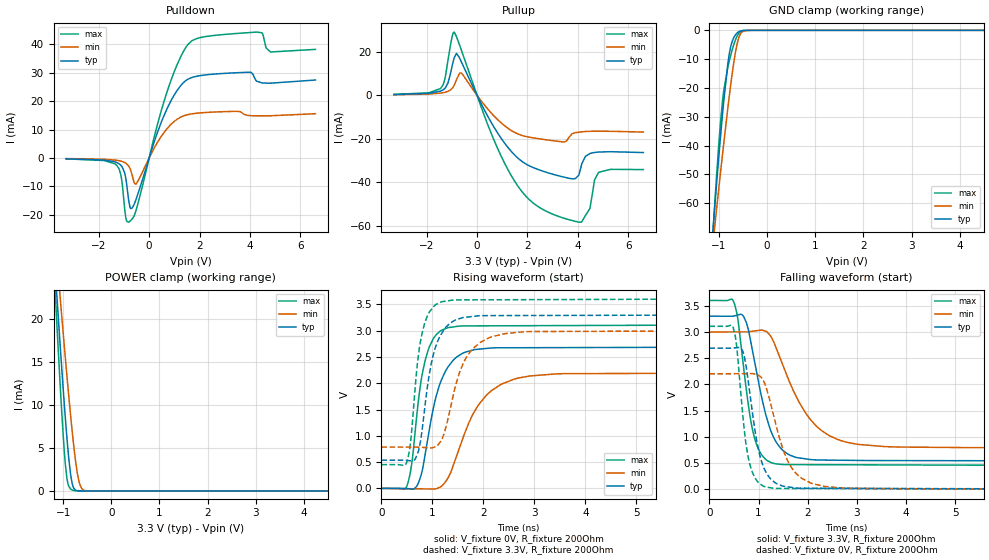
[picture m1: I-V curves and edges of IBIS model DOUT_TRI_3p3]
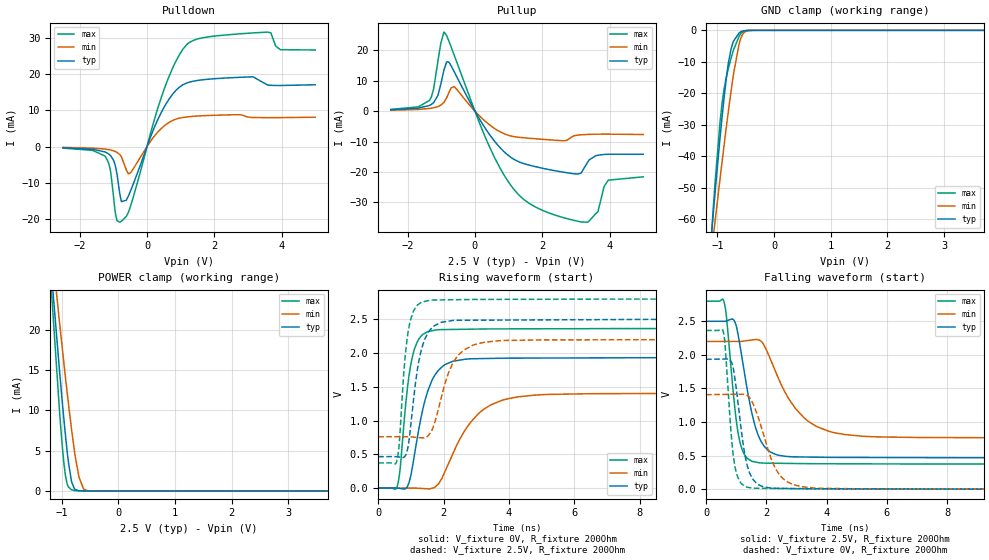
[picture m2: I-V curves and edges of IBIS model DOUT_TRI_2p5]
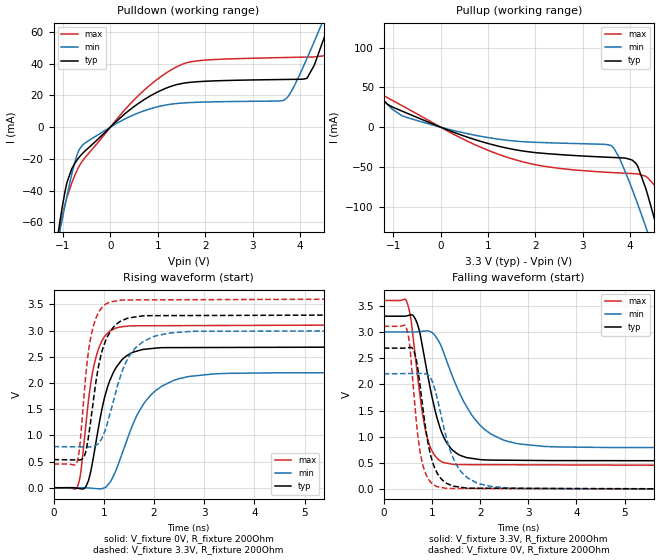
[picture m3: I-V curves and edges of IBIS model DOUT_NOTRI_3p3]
|Texas Instruments Incorporated
| Marketing part#   Digital Voltage Range   Package-type   #pins
| ADS1287D   2.2V - 3.6V   VQFN   32
[IBIS Ver]   4.1
[File name]   ads1287d.ibs
[File Rev]   1.0
[Date]   03/20/2017
[Source]
| Texas Instruments Incorporated.
| 12500 TI Blvd
| Dallas, TX -75243
[Notes]   Revision History:
| Rev 1.0: 03/20/2017
| - Initial version of the model
| - Model generated from simulations in TISPICE
| - C_comp although listed in numerical order of value are
|   obtained from varying PVT conditions. For PVT conditions for
|   each specific value refer the buffer description under
|   respective [Model]. IBIS model user is responsible for using
|   appropriate C_comp to simulate for Signal Integrity.
| - Warnings regarding combined Non-monotonicity of various models have been
|   reviewd and considered minor and can be ignored.
| - Model names with a trailing _2p5 contain the model for
|   2.5V operation. Model names with a trailing _3p3 contain the model
|   for 3.3V operation.
[Disclaimer]
| This model is designed as an aid for customers of Texas Instruments.
| TI and its licensors and suppliers make no warranties, either expressed
| or implied, with respect to this  model, including the warranties of
| merchantability or fitness for a particular purpose. The model is
| provided solely on an "as is" basis. The entire risk as to its quality
| and performance is with the customer.
[Copyright]
 (C) Copyright 2016 Texas Instruments Incorporated.All rights reserved.
|   Device
[Component]  ADS1287D
[Manufacturer]   TI
[Package]
| variable   typ   min   max
R_pkg   0.01   0.008   0.012
L_pkg   0.1nH   0.08nH   0.12nH
C_pkg   0.1pF   0.08pF   0.12pF
[Pin]  signal_name   model_name   R_pin   L_pin   C_pin
1   DRDY2\   DOUT_NOTRI   NA   NA   NA
2   DOUT   DOUT_TRI   NA   NA   NA
3   DIN   DIN   NA   NA   NA
4   CS1\   DIN   NA   NA   NA
5   CS2\   DIN   NA   NA   NA
6   SYNC   DIN   NA   NA   NA
7   TCP1   DIO   NA   NA   NA
8   TCP2   DIO   NA   NA   NA
9   CAPN1   NC   NA   NA   NA
10   CAPP1   NC   NA   NA   NA
11   CAPN2   NC   NA   NA   NA
12   CAPP2   NC   NA   NA   NA
13   TCR1   NC   NA   NA   NA
14   TCR2   NC   NA   NA   NA
15   AINP1   NC   NA   NA   NA
16   AINN1   NC   NA   NA   NA
17   AINP2   NC   NA   NA   NA
18   AINN2   NC   NA   NA   NA
19   AVDD   POWER   NA   NA   NA
20   AVSS   GND   NA   NA   NA
21   REFN   NC   NA   NA   NA
22   REFP   NC   NA   NA   NA
23   PWDN1\   DIN   NA   NA   NA
24   PWDN2\   DIN   NA   NA   NA
25   RESET\   DIN   NA   NA   NA
26   DVDD   POWER   NA   NA   NA
27   DGND   GND   NA   NA   NA
28   BYPAS1   NC   NA   NA   NA
29   BYPAS2   NC   NA   NA   NA
30   CLK   DIN_PD   NA   NA   NA
31   SCLK   DIN_PD   NA   NA   NA
32   DRDY1\   DOUT_NOTRI   NA   NA   NA
|   Model Selectors
[Model Selector]  DIN
DIN_3p3  input buffer at 3.3V operation.
DIN_2p5  input buffer at 2.5V operation.
[Model Selector]  DIN_PD
DIN_PD_3p3  input buffer at 3.3V operation.
DIN_PD_2p5  input buffer at 2.5V operation.
[Model Selector]  DIO
DIO_3p3  output buffer at 3.3V operation.
DIO_2p5  output buffer at 2.5V operation.
[Model Selector]  DOUT_TRI
DOUT_TRI_3p3  output buffer at 3.3V operation.
DOUT_TRI_2p5  output buffer at 2.5V operation.
[Model Selector]  DOUT_NOTRI
DOUT_NOTRI_3p3  output buffer at 3.3V operation.
DOUT_NOTRI_2p5  output buffer at 2.5V operation.
| Models and submodels in the file (10): DOUT_TRI_3p3 (3-state), DOUT_TRI_2p5 (3-state), DOUT_NOTRI_3p3 (Output), DOUT_NOTRI_2p5 (Output), DIO_3p3 (I/O), DIO_2p5 (I/O), DIN_PD_3p3 (Input), DIN_PD_2p5 (Input), DIN_3p3 (Input), DIN_2p5 (Input)
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|   Model
[Model]   DOUT_TRI_3p3
Model_type   3-state
Polarity   Non-Inverting
Vmeas = 1.65
Vref = 0
Cref = 1pF
Rref = 100000
|   typ   min   max
C_comp   3.353pF   2.933pF   3.722pF
[Voltage Range]   3.3   3   3.6
[Temperature Range]   27   125   -40
[Pullup Reference]   3.3   3   3.6
[Pulldown Reference]   0   0   -0
[Power Clamp Reference]   3.3   3   3.6
[GND Clamp Reference]   0   0   0
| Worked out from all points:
|   slope of the pulldown table from 0 to 0.495 V, typ, clamps not added: 38.4 ohm
|   slope of the pullup table from 0 to 0.495 V, typ, clamps not added: 44.6 ohm
|   GND clamp passes 1 mA (typ) near -0.63 V on its own axis
|   POWER clamp passes 1 mA (typ) near -0.82 V on its own axis
|   falling waveform, V_fixture 3.3V, R_fixture 200Ohm: 20-80 % time 405ps typ, 736ps min, 275ps max; typ from 3.3 V to 0.537 V
|   rising waveform, V_fixture 0V, R_fixture 200Ohm: 20-80 % time 381ps typ, 640ps min, 259ps max; typ from 0 V to 2.69 V
|   rising waveform, V_fixture 3.3V, R_fixture 200Ohm: 20-80 % time 288ps typ, 429ps min, 211ps max; typ from 0.537 V to 3.3 V
|   falling waveform, V_fixture 0V, R_fixture 200Ohm: 20-80 % time 282ps typ, 440ps min, 207ps max; typ from 2.69 V to 0 V
[Pulldown]
|   Voltage   I(typ)   I(min)   I(max)
-3.3V     -275.6uA   -195.7uA   -299.2uA
-1.29V    -1.589mA   -812uA     -2.567mA
-1.112V   -2.674mA   -1.126mA   -6.407mA
-973.5mV  -5.243mA   -1.59mA    -17.68mA
-815.1mV  -14.85mA   -2.806mA   -22.59mA
-726mV    -17.84mA   -4.463mA   -21.94mA
-518.1mV  -14.5mA    -9.108mA   -18.41mA
709.5mV   17.33mA    10.32mA    23.26mA
1.68V     28.27mA    15.51mA    41.13mA
4.274V    27.01mA    14.85mA    44.32mA
4.818V    26.34mA    14.87mA    37.31mA
6.6V      27.45mA    15.59mA    38.23mA
[GND Clamp]
|   Voltage   I(typ)   I(min)   I(max)
-3.3V     -596mA     -481.9mA   -706.9mA
-1.191V   -83.7mA    -85.04mA   -87.73mA
-1.092V   -62.16mA   -68.77mA   -61.24mA
-1.063V   -55.89mA   -64.02mA   -53.64mA
-983.4mV  -39.78mA   -51.67mA   -34.99mA
-904.2mV  -25.08mA   -39.7mA    -21.25mA
-815.1mV  -11.44mA   -26.82mA   -12.68mA
-755.7mV  -5.637mA   -18.79mA   -8.611mA
-656.7mV  -1.555mA   -7.52mA    -3.281mA
-567.6mV  -310.1uA   -1.686mA   -686.5uA
-280.5mV  -30.52nA   -1.575uA   -574.7nA
6.6V      0A         0A         0A
[Pullup]
|   Voltage   I(typ)   I(min)   I(max)
-3.3V     367.9uA    267.7uA    426.7uA
-1.439V   1.996mA    1.043mA    3.259mA
-1.162V   5.477mA    1.816mA    15.57mA
-914.1mV  17.05mA    4.508mA    29.15mA
-617.1mV  15.27mA    10.17mA    20.63mA
986.7mV   -20.32mA   -13mA      -28.77mA
2.373V    -33.95mA   -19.86mA   -50.87mA
3.769V    -38.49mA   -17.71mA   -57.69mA
4.125V    -33.01mA   -16.86mA   -58.46mA
4.471V    -26.85mA   -16.59mA   -52.31mA
4.818V    -26.14mA   -16.53mA   -35.56mA
6.6V      -26.37mA   -16.92mA   -34.22mA
[POWER Clamp]
|   Voltage   I(typ)   I(min)   I(max)
-3.3V     222.9mA    184.2mA    273.8mA
-1.181V   27.13mA    30.69mA    24.94mA
-1.122V   22.01mA    26.62mA    18.54mA
-1.063V   17.02mA    22.61mA    12.42mA
-1.003V   12.21mA    18.66mA    6.83mA
-953.7mV  8.435mA    15.45mA    3.071mA
-904.2mV  5.034mA    12.34mA    929.6uA
-844.8mV  1.889mA    8.78mA     223.7uA
-805.2mV  702.8uA    6.57mA     94.47uA
-676.5mV  12.39uA    1.245mA    3.073uA
-528mV    121.8nA    27.64uA    0A
6.6V      0A         0A         0A
[Ramp]
R_load = 200
|   typ   min   max
dV/dt_r   1.61412/3.77044e-10   1.32022/6.35916e-10   1.86431/2.58199e-10
dV/dt_f   1.65772/4.03606e-10   1.32906/7.34637e-10   1.88895/2.74389e-10
[Falling Waveform]
V_fixture = 3.3V
V_fixture_min = 3V
V_fixture_max = 3.6V
R_fixture = 200Ohm
C_fixture = 0F
|   Time   V(typ)   V(min)   V(max)
0s        3.3V       3V         3.6V
490.8ps   3.301V     3V         3.583V
696.4ps   3.296V     3V         2.328V
829.8ps   2.875V     3.007V     1.381V
966.6ps   2.208V     3.024V     838.8mV
1.218ns   1.199V     2.954V     525.5mV
1.464ns   769.1mV    2.442V     471.8mV
2.281ns   555.1mV    1.118V     466.8mV
3.566ns   545.6mV    812.4mV    463.2mV
50ns      537.1mV    784.9mV    451.7mV
[Rising Waveform]
V_fixture = 0V
V_fixture_min = 0V
V_fixture_max = 0V
R_fixture = 200Ohm
C_fixture = 0F
|   Time   V(typ)   V(min)   V(max)
0s        -237.1nV   -255.9nV   -93.79nV
490.8ps   -2.67mV    -5.275mV   28.16mV
594.8ps   -11.92mV   -6.392mV   472.9mV
696.4ps   50.2mV     -7.484mV   1.418V
946.5ps   1.156V     -10.17mV   2.708V
1.172ns   2.054V     38.1mV     3.003V
1.525ns   2.53V      758.1mV    3.086V
2.164ns   2.67V      1.863V     3.091V
3.566ns   2.677V     2.182V     3.096V
50ns      2.69V      2.2V       3.107V
[Rising Waveform]
V_fixture = 3.3V
V_fixture_min = 3V
V_fixture_max = 3.6V
R_fixture = 200Ohm
C_fixture = 0F
|   Time   V(typ)   V(min)   V(max)
0s        537.1mV    784.9mV    451.7mV
490.8ps   533mV      785.1mV    486mV
574.3ps   525mV      785.2mV    912.4mV
666.4ps   562.7mV    785.2mV    1.975V
908.3ps   1.979V     773.8mV    3.295V
1.172ns   2.932V     906.5mV    3.544V
1.407ns   3.18V      1.765V     3.582V
1.802ns   3.271V     2.666V     3.585V
2.901ns   3.287V     2.982V     3.589V
50ns      3.3V       3V         3.6V
[Falling Waveform]
|Gnd
V_fixture = 0V
V_fixture_min = 0V
V_fixture_max = 0V
R_fixture = 200Ohm
C_fixture = 0F
|   Time   V(typ)   V(min)   V(max)
0s        2.69V      2.2V       3.107V
482ps     2.692V     2.203V     3.09V
553.5ps   2.699V     2.203V     2.744V
666.4ps   2.658V     2.203V     1.554V
873.1ps   1.484V     2.204V     326.2mV
1.052ns   558.8mV    2.137V     87.07mV
1.303ns   148.5mV    1.421V     16.29mV
1.767ns   21.14mV    296.3mV    13.28mV
2.791ns   15.52mV    19.55mV    11.12mV
50ns      -231.5nV   -246.5nV   -88.11nV
|   Model
[Model]   DOUT_TRI_2p5
Model_type   3-state
Polarity   Non-Inverting
Vmeas = 1.25
Vref = 0
Cref = 1pF
Rref = 100000
|   typ   min   max
C_comp   3.353pF   2.933pF   3.722pF
[Voltage Range]   2.5   2.2   2.8
[Temperature Range]   27   125   -40
[Pullup Reference]   2.5   2.2   2.8
[Pulldown Reference]   0   0   0
[Power Clamp Reference]   2.5   2.2   2.8
[GND Clamp Reference]   0   0   0
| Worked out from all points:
|   slope of the pulldown table from 0 to 0.375 V, typ, clamps not added: 44.2 ohm
|   slope of the pullup table from 0 to 0.375 V, typ, clamps not added: 55.4 ohm
|   GND clamp passes 1 mA (typ) near -0.62 V on its own axis
|   POWER clamp passes 1 mA (typ) near -0.82 V on its own axis
|   falling waveform, V_fixture 2.5V, R_fixture 200Ohm: 20-80 % time 532ps typ, 1.13ns min, 325ps max; typ from 2.5 V to 0.466 V
|   rising waveform, V_fixture 0V, R_fixture 200Ohm: 20-80 % time 532ps typ, 1.05ns min, 317ps max; typ from 0 V to 1.93 V
|   rising waveform, V_fixture 2.5V, R_fixture 200Ohm: 20-80 % time 365ps typ, 589ps min, 244ps max; typ from 0.466 V to 2.5 V
|   falling waveform, V_fixture 0V, R_fixture 200Ohm: 20-80 % time 359ps typ, 651ps min, 240ps max; typ from 1.93 V to 0 V
[Pulldown]
|   Voltage   I(typ)   I(min)   I(max)
-2.5V     -352.9uA   -224.1uA   -417.5uA
-1.24V    -1.522mA   -700.3uA   -2.753mA
-1.105V   -2.303mA   -904.7uA   -5.819mA
-977.5mV  -4.208mA   -1.237mA   -15.49mA
-812.5mV  -12.83mA   -2.205mA   -20.85mA
-760mV    -15.19mA   -2.847mA   -20.57mA
-512.5mV  -12.74mA   -7.386mA   -17.06mA
522.5mV   11.12mA    5.789mA    16.17mA
1.212V    17.64mA    8.204mA    28.38mA
3.583V    16.97mA    7.969mA    31.57mA
3.965V    16.85mA    7.987mA    26.71mA
5V        17.04mA    8.093mA    26.63mA
[GND Clamp]
|   Voltage   I(typ)   I(min)   I(max)
-2.5V     -397mA     -325.5mA   -469.1mA
-1.232V   -92.88mA   -91.97mA   -99.09mA
-1.067V   -56.92mA   -64.8mA    -54.88mA
-1.052V   -53.78mA   -62.42mA   -51.11mA
-955mV    -34.31mA   -47.33mA   -29.29mA
-917.5mV  -27.42mA   -41.69mA   -23.07mA
-805mV    -10.22mA   -25.41mA   -11.94mA
-715mV    -3.396mA   -13.75mA   -6.179mA
-617.5mV  -825.6uA   -4.302mA   -1.836mA
-580mV    -402.8uA   -2.177mA   -901.3uA
-347.5mV  -745.5nA   -9.998uA   -541.4nA
5V        0A         0A         0A
[Pullup]
|   Voltage   I(typ)   I(min)   I(max)
-2.5V     456.2uA    297.4uA    576.9uA
-1.353V   1.877mA    880.3uA    3.514mA
-1.105V   5.099mA    1.503mA    16.08mA
-917.5mV  13.7mA     2.98mA     26.01mA
-617.5mV  12.99mA    8.073mA    18.45mA
537.5mV   -9.248mA   -5.346mA   -14.22mA
1.482V    -17.34mA   -8.776mA   -29.31mA
3.058V    -20.66mA   -7.85mA    -36.2mA
3.35V     -16.78mA   -7.653mA   -36.52mA
3.658V    -14.49mA   -7.57mA    -32.96mA
3.965V    -14.16mA   -7.561mA   -22.69mA
5V        -14.19mA   -7.674mA   -21.6mA
[POWER Clamp]
|   Voltage   I(typ)   I(min)   I(max)
-2.5V     148mA      125.5mA    178.6mA
-1.188V   27.66mA    31.11mA    25.61mA
-1.038V   14.96mA    20.93mA    9.967mA
-962.5mV  9.084mA    16.02mA    3.644mA
-932.5mV  6.919mA    14.11mA    1.918mA
-902.5mV  4.927mA    12.23mA    889.1uA
-827.5mV  1.271mA    7.794mA    154.1uA
-775mV    282uA      5.012mA    46.54uA
-692.5mV  20.27uA    1.675mA    4.969uA
-617.5mV  2.149uA    323.3uA    451.7nA
-550mV    278.9nA    51.46uA    15.26nA
5V        0A         0A         0A
[Ramp]
R_load = 200
|   typ   min   max
dV/dt_r   1.15988/5.28506e-10   0.84445/1.04064e-09   1.41824/3.16387e-10
dV/dt_f   1.22037/5.31867e-10   0.863307/1.13119e-09   1.45603/3.24917e-10
[Falling Waveform]
V_fixture = 2.5V
V_fixture_min = 2.2V
V_fixture_max = 2.8V
R_fixture = 200Ohm
C_fixture = 0F
|   Time   V(typ)   V(min)   V(max)
0s        2.5V       2.2V       2.8V
608.6ps   2.5V       2.2V       2.765V
959.2ps   2.485V     2.2V       1.185V
1.215ns   1.891V     2.204V     567.8mV
1.512ns   1.145V     2.221V     415.9mV
1.76ns    770.2mV    2.22V      392.5mV
2.283ns   521.3mV    1.775V     385.9mV
3.239ns   478.9mV    1.067V     380.6mV
5.234ns   471.8mV    787.2mV    376.9mV
50ns      466.1mV    761.2mV    373.3mV
[Rising Waveform]
V_fixture = 0V
V_fixture_min = 0V
V_fixture_max = 0V
R_fixture = 200Ohm
C_fixture = 0F
|   Time   V(typ)   V(min)   V(max)
0s        -482.1nV   -1.004uV   -83.95nV
585.7ps   219.1uV    125.3uV    33.95mV
669.6ps   -4.751mV   143.4uV    279.2mV
898.3ps   28.26mV    192.7uV    1.498V
1.183ns   708.9mV    -632.4uV   2.153V
1.452ns   1.336V     -8.438mV   2.301V
1.76ns    1.691V     25.14mV    2.342V
3.05ns    1.918V     1.095V     2.356V
4.799ns   1.926V     1.378V     2.36V
50ns      1.933V     1.407V     2.364V
[Rising Waveform]
V_fixture = 2.5V
V_fixture_min = 2.2V
V_fixture_max = 2.8V
R_fixture = 200Ohm
C_fixture = 0F
|   Time   V(typ)   V(min)   V(max)
0s        466.1mV    761.2mV    373.3mV
563.7ps   465.2mV    761.1mV    388.7mV
645.8ps   460.3mV    761.1mV    671.5mV
856.3ps   503.5mV    761.1mV    2.092V
991.4ps   910.2mV    759.4mV    2.494V
1.241ns   1.874V     749.1mV    2.726V
1.568ns   2.331V     799.7mV    2.782V
2.378ns   2.486V     1.923V     2.791V
3.675ns   2.489V     2.182V     2.795V
50ns      2.5V       2.2V       2.8V
[Falling Waveform]
|Gnd
V_fixture = 0V
V_fixture_min = 0V
V_fixture_max = 0V
R_fixture = 200Ohm
C_fixture = 0F
|   Time   V(typ)   V(min)   V(max)
0s        1.933V     1.407V     2.364V
563.7ps   1.937V     1.411V     2.356V
639.2ps   1.938V     1.411V     2.085V
856.3ps   1.877V     1.412V     687.3mV
1.084ns   1.188V     1.414V     143.6mV
1.309ns   459.2mV    1.408V     38.57mV
1.514ns   178.6mV    1.312V     17.39mV
2.42ns    12.36mV    221.9mV    9.884mV
3.558ns   6.242mV    17.95mV    4.962mV
50ns      -503.2nV   -992.2nV   -79.5nV
|   Model
[Model]   DOUT_NOTRI_3p3
Model_type   Output
Polarity   Non-Inverting
Vmeas = 1.65
Vref = 0
Cref = 1pF
Rref = 100000
|   typ   min   max
C_comp   3.353pF   2.933pF   3.722pF
[Voltage Range]   3.3   3   3.6
[Temperature Range]   27   125   -40
[Pullup Reference]   3.3   3   3.6
[Pulldown Reference]   -0   0   0
[Power Clamp Reference]   3.3   3   3.6
[GND Clamp Reference]   0   0   0
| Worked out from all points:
|   slope of the pulldown table from 0 to 0.495 V, typ, clamps not added: 38.5 ohm
|   slope of the pullup table from 0 to 0.495 V, typ, clamps not added: 44.5 ohm
|   falling waveform, V_fixture 3.3V, R_fixture 200Ohm: 20-80 % time 402ps typ, 730ps min, 275ps max; typ from 3.3 V to 0.537 V
|   rising waveform, V_fixture 0V, R_fixture 200Ohm: 20-80 % time 384ps typ, 644ps min, 262ps max; typ from 0 V to 2.69 V
|   rising waveform, V_fixture 3.3V, R_fixture 200Ohm: 20-80 % time 301ps typ, 470ps min, 215ps max; typ from 0.537 V to 3.3 V
|   falling waveform, V_fixture 0V, R_fixture 200Ohm: 20-80 % time 278ps typ, 423ps min, 208ps max; typ from 2.69 V to 0 V
[Pulldown]
|   Voltage   I(typ)   I(min)   I(max)
-3.3V     -596.3mA   -482.1mA   -707.2mA
-1.063V   -59.16mA   -65.28mA   -63.1mA
-914.1mV  -34.7mA    -43.09mA   -44.08mA
-587.4mV  -16.59mA   -11.34mA   -21.23mA
570.9mV   14.54mA    8.755mA    19.35mA
1.541V    27.73mA    15.28mA    39.96mA
3.67V     30.09mA    17.11mA    43.95mA
4.155V    31.06mA    43.71mA    44.25mA
4.561V    60.46mA    72.23mA    45.2mA
4.709V    73.7mA     82.88mA    55mA
5.273V    125.5mA    123.9mA    118.2mA
6.6V      250.4mA    221.9mA    276.3mA
[Pullup]
|   Voltage   I(typ)   I(min)   I(max)
-3.3V     223.3mA    184.5mA    274.2mA
-1.409V   49.5mA     47.7mA     54.22mA
-1.122V   28.89mA    28.64mA    37.07mA
-815.1mV  20.24mA    14.32mA    27.13mA
1.403V    -26.42mA   -16.52mA   -37.87mA
3.59V     -38.06mA   -23.1mA    -57.12mA
3.769V    -38.52mA   -38.19mA   -57.69mA
4.125V    -45.73mA   -90.93mA   -58.7mA
4.333V    -77.5mA    -125.8mA   -61.95mA
4.561V    -125.7mA   -165.9mA   -77.13mA
4.808V    -182.5mA   -211mA     -128mA
6.6V      -622.3mA   -558.3mA   -651.8mA
[Ramp]
R_load = 200
|   typ   min   max
dV/dt_r   1.61412/3.81689e-10   1.32022/6.43462e-10   1.86431/2.61812e-10
dV/dt_f   1.65772/4.01795e-10   1.32905/7.29868e-10   1.88895/2.74388e-10
[Falling Waveform]
V_fixture = 3.3V
V_fixture_min = 3V
V_fixture_max = 3.6V
R_fixture = 200Ohm
C_fixture = 0F
|   Time   V(typ)   V(min)   V(max)
0s        3.3V       3V         3.6V
473.2ps   3.305V     3V         3.589V
667.7ps   3.226V     2.999V     2.439V
811.3ps   2.684V     3.013V     1.402V
953.1ps   1.982V     3.009V     835.1mV
1.192ns   1.11V      2.732V     530.7mV
1.452ns   727.3mV    2.094V     471.7mV
2.236ns   554.9mV    1.046V     466.7mV
3.651ns   545.1mV    804.9mV    462.6mV
50ns      537.1mV    784.9mV    451.7mV
[Rising Waveform]
V_fixture = 0V
V_fixture_min = 0V
V_fixture_max = 0V
R_fixture = 200Ohm
C_fixture = 0F
|   Time   V(typ)   V(min)   V(max)
0s        -16.67nV   -219.2nV   -183.6nV
473.2ps   -9.407mV   585.3uV    14.06mV
641ps     15.51mV    -480.4uV   1.172V
752.8ps   366.8mV    -8.73mV    2.069V
913.8ps   1.248V     -20.61mV   2.697V
1.121ns   2.046V     101.5mV    2.988V
1.513ns   2.551V     1.046V     3.087V
2.166ns   2.672V     1.945V     3.092V
3.486ns   2.677V     2.183V     3.096V
50ns      2.69V      2.2V       3.107V
[Rising Waveform]
V_fixture = 3.3V
V_fixture_min = 3V
V_fixture_max = 3.6V
R_fixture = 200Ohm
C_fixture = 0F
|   Time   V(typ)   V(min)   V(max)
0s        537.1mV    784.9mV    451.7mV
464.7ps   530.8mV    781mV      482.8mV
614.5ps   606.2mV    779.7mV    1.842V
720.6ps   1.139V     778.8mV    2.758V
841.2ps   2.001V     808.7mV    3.228V
1.036ns   2.804V     1.119V     3.499V
1.342ns   3.182V     2.153V     3.58V
1.781ns   3.279V     2.786V     3.584V
2.803ns   3.286V     2.985V     3.588V
50ns      3.3V       3V         3.6V
[Falling Waveform]
|Gnd
V_fixture = 0V
V_fixture_min = 0V
V_fixture_max = 0V
R_fixture = 200Ohm
C_fixture = 0F
|   Time   V(typ)   V(min)   V(max)
0s        2.69V      2.2V       3.107V
464.7ps   2.694V     2.204V     3.095V
614.5ps   2.661V     2.206V     1.947V
708.7ps   2.293V     2.206V     1.018V
825ps     1.463V     2.206V     417.2mV
998.1ps   564.5mV    2.077V     111.3mV
1.291ns   120.3mV    1.012V     16.14mV
1.748ns   19.57mV    210.9mV    13.18mV
2.803ns   15.35mV    15.83mV    10.88mV
50ns      -231.8nV   -204.6nV   -76.9nV
